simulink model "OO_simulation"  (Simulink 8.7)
settings: Solver=ode45  StartTime=0.0  StopTime=2000  RelTol=1e-3
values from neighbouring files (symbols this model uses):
  Ao = Am - Ko * Cm    [OO_design.m]
  Bo = [Bm Ko]    [OO_design.m]
  Co = Cm    [OO_design.m]
  Do = zeros(1,2)    [OO_design.m]
  Ts = 0.2    [init_model.m]

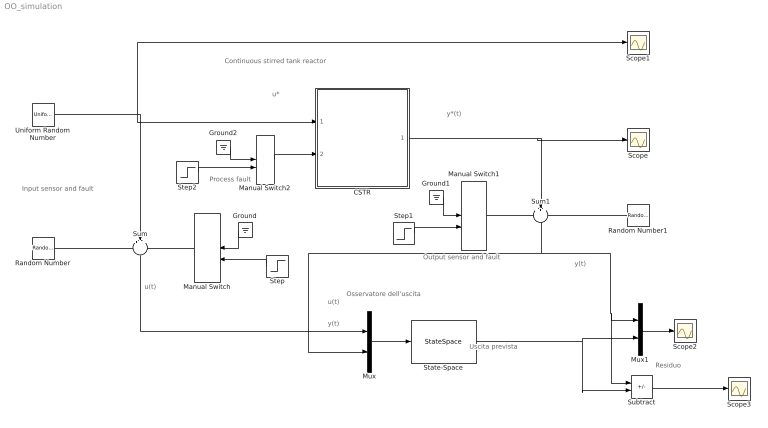
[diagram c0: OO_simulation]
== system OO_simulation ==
  note: Residuo
  note: Uscita prevista
  note: Osservatore dell'uscita
  note: y(t)
  note: u(t)
  note: y(t)
  note: y*(t)
  note: u*
  note: Continuous stirred tank reactor
  note: Process fault
  note: Input sensor and fault
  note: Output sensor and fault
  note: u(t)
  CSTR : Subsystem
  Ground : Ground
  Ground1 : Ground
  Ground2 : Ground
  Manual Switch : ManualSwitch
  Manual Switch1 : ManualSwitch
  Manual Switch2 : ManualSwitch
  Mux : Mux  Inputs=2
  Mux1 : Mux  Inputs=2
  Random Number : RandomNumber  Variance=0.0001  Seed=1  SampleTime=Ts
  Random Number1 : RandomNumber  Variance=0.0001  Seed=2  SampleTime=Ts
  Scope{,1..3} (4 alike) : Scope
  State-Space : StateSpace  A=Ao  B=Bo  C=Co  D=Do  X0=0
  Step : Step  Time=1000  After=10  SampleTime=0
  Step1 : Step  Time=1000  After=10  SampleTime=0
  Step2 : Step  Time=1000  SampleTime=0
  Subtract : Sum  Inputs=+-
  Sum : Sum  Inputs=+++  SaturateOnIntegerOverflow=on
  Sum1 : Sum  Inputs=+++  SaturateOnIntegerOverflow=on
  Uniform Random Number : UniformRandomNumber  Minimum=0  Maximum=4  SampleTime=20
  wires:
  Uniform Random Number/1 -> Sum/2, CSTR/1(w), Scope1/1
  Random Number/1 -> Sum/1
  Manual Switch/1 -> Sum/3
  Sum/1 -> Mux/1
  Ground/1 -> Manual Switch/1
  Step/1 -> Manual Switch/2
  Ground1/1 -> Manual Switch1/1
  Step1/1 -> Manual Switch1/2
  CSTR/1(Cb) -> Sum1/2, Scope/1
  Sum1/1 -> Subtract/1, Mux1/1, Mux/2
  Manual Switch1/1 -> Sum1/1
  Random Number1/1 -> Sum1/3
  Step2/1 -> Manual Switch2/2
  Ground2/1 -> Manual Switch2/1
  Manual Switch2/1 -> CSTR/2(f)
  Mux/1 -> State-Space/1
  State-Space/1 -> Subtract/2, Mux1/2
  Mux1/1 -> Scope2/1
  Subtract/1 -> Scope3/1

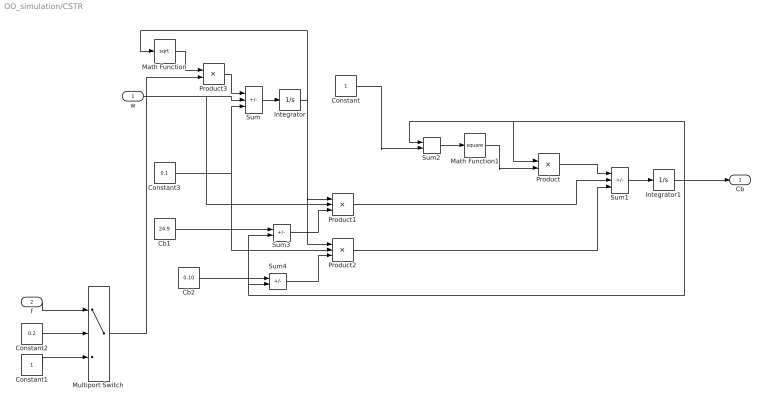
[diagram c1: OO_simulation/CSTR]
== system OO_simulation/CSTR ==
  w : Inport
  f : Inport  Port=2
  Cb1 : Constant  Value=24.9
  Cb2 : Constant  Value=0.10
  Constant : Constant
  Constant1 : Constant
  Constant2 : Constant  Value=0.2
  Constant3 : Constant  Value=0.1
  Integrator : Integrator  InitialCondition=30  LimitOutput=on  LowerSaturationLimit=1
  Integrator1 : Integrator  InitialCondition=22
  Math Function : Math  Operator=sqrt
  Math Function1 : Math  Operator=square
  Multiport Switch : MultiPortSwitch  DataPortOrder=Zero-based contiguous  Inputs=2  zeroidx=on
  Product : Product  Inputs=*/  SaturateOnIntegerOverflow=on
  Product1 : Product  Inputs=/**  SaturateOnIntegerOverflow=on
  Product2 : Product  Inputs=/**  SaturateOnIntegerOverflow=on
  Product3 : Product
  Sum : Sum  Inputs=-++  SaturateOnIntegerOverflow=on
  Sum1 : Sum  Inputs=-++  SaturateOnIntegerOverflow=on
  Sum2 : Sum  SaturateOnIntegerOverflow=on
  Sum3 : Sum  Inputs=+-  SaturateOnIntegerOverflow=on
  Sum4 : Sum  Inputs=+-  SaturateOnIntegerOverflow=on
  Cb : Outport
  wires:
  Sum/1 -> Integrator/1
  Product3/1 -> Sum/1
  Math Function/1 -> Product3/1
  Integrator/1 -> Math Function/1, Product1/1, Product2/1
  Sum3/1 -> Product1/3
  Sum4/1 -> Product2/3
  Sum2/1 -> Math Function1/1
  Sum1/1 -> Integrator1/1
  Math Function1/1 -> Product/2
  Product/1 -> Sum1/1
  Product1/1 -> Sum1/2
  Product2/1 -> Sum1/3
  w/1 -> Sum/2, Product1/2
  Constant3/1 -> Product2/2, Sum/3
  Integrator1/1 -> Sum3/2, Sum4/2, Sum2/1, Product/1, Cb/1
  Constant1/1 -> Multiport Switch/3
  f/1 -> Multiport Switch/1
  Constant2/1 -> Multiport Switch/2
  Cb2/1 -> Sum4/1
  Cb1/1 -> Sum3/1
  Constant/1 -> Sum2/2
  Multiport Switch/1 -> Product3/2
